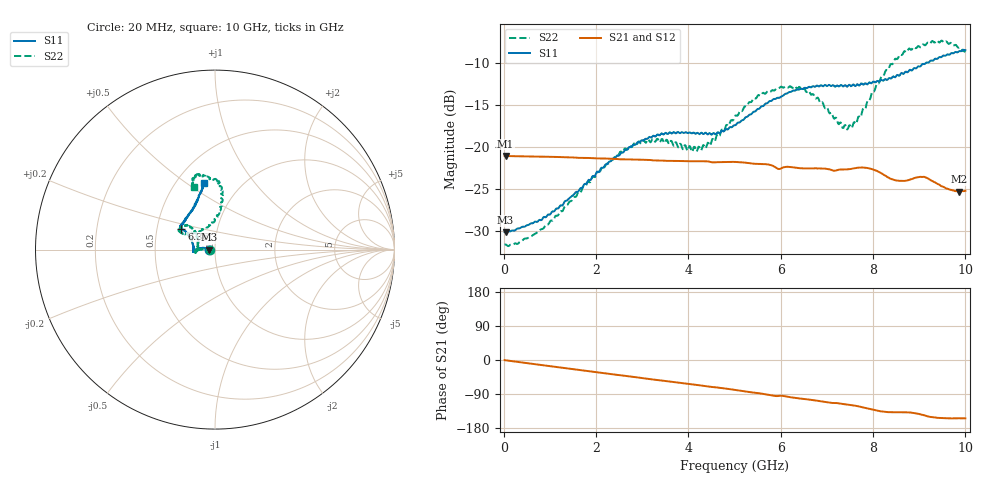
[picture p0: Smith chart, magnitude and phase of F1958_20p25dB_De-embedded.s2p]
! Integrated Device Technology
! Corporate Headquarters
! 6024 Silver Creek Valley Road
! San Jose, CA 95138  USA
! Phone:  1-408-284-8200
! Toll Free:  1-800-223-1366
! Webpage:  http://www.idt.com/
! Timing and RF Division
! 515 Groton Road, Suite 102
! Westford, MA 01886-6024
! Device:  F1958
! Description: 7-bit 0.25 dB Digital Step Attenuator
! Frequency:  0.001 -  6.000 GHz
! Package:  4x4 mm Thin QFN Plastic Package: 24 pin
! Ports:  2 RF, 12 DC
!  Pin  1  = D0
!  Pin  2  = VDD
!  Pin  3  = VMODE
!  Pin  4  = GND
!  Pin  5  = RF1  =  Port 1
!  Pin  6  = GND
!  Pin  7  = GND
!  Pin  8  = GND
!  Pin  9  = GND
!  Pin 10  = GND
!  Pin 11  = GND
!  Pin 12  = GND
!  Pin 13  = GND
!  Pin 14  = RF2  =  Port 2
!  Pin 15  = GND
!  Pin 16  = LE
!  Pin 17  = CLK
!  Pin 18  = DATA
!  Pin 19  = D6
!  Pin 20  = D5
!  Pin 21  = D4
!  Pin 22  = D3
!  Pin 23  = D2
!  Pin 24  = D1
! State:  81
! Atten State:  20.25 dB
! Voltage:  +3.30 Volts
! Current:  0.258 mA
! Data:  The device was measured on a F1958 evaluation board which has
!  individual transmission lines to the RF pins.  Data was collected
!  using a calibrated network analyzer.  The evaluation board was
!  de-embedded using Automatic Fixture Removal (AFR).
!  The reference plane is the edge of the package pin.
! Misc:
!  Action Tracker AT0419
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# GHz S dB R 50
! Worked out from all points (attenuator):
!   500 points, 20 MHz to 10 GHz, reference 50 ohm
!   highest |S21| = -21.03 dB at 40 MHz (marker M1); lowest = -25.3 dB at 9.86 GHz (marker M2)
!   lowest |S11| = -30.1 dB at 40 MHz (marker M3), VSWR 1.06, Z = 47 - j0.0438 ohm
!   |S11| at or under -10 dB: start of sweep to 9.139 GHz
!   |S22| runs from -31.7 to -7.3 dB; largest |S21 - S12| = 0.00031
!   S11 on the Smith chart (normalised r, x): 20 MHz: 0.94, -0.00; 6.36 GHz: 0.67, +0.16; 10 GHz: 0.67, +0.59
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0.02  -30.06 -178.9  -21.03 -0.4  -21.03 -0.4  -31.57 -178.6
0.04  -30.10 -179.1  -21.03 -0.7  -21.02 -0.7  -31.53 -177.9
0.32  -29.63 175.2  -21.06 -5.3  -21.06 -5.3  -31.40 177.6
0.84  -28.50 171.1  -21.11 -13.6  -21.11 -13.6  -29.70 178.0
1.7  -24.81 171.3  -21.26 -27.2  -21.25 -27.2  -24.91 176.6
2.62  -20.36 177.4  -21.42 -41.6  -21.40 -41.6  -20.15 -177.8
3.36  -18.56 -175.5  -21.58 -53.3  -21.57 -53.4  -19.27 -171.1
4.24  -18.44 -179.0  -21.65 -66.7  -21.66 -66.8  -19.96 166.7
4.64  -18.20 171.9  -21.77 -72.8  -21.78 -72.8  -18.49 148.6
5.02  -17.37 160.9  -21.74 -79.1  -21.75 -79.1  -16.21 138.1
5.58  -15.13 150.7  -21.99 -88.6  -22.00 -88.6  -13.78 138.4
6.36  -13.12 148.0  -22.44 -100.8  -22.46 -100.7  -13.04 151.5
6.68  -12.78 146.5  -22.50 -105.5  -22.52 -105.4  -13.72 152.4
7.3  -12.59 140.8  -22.64 -115.1  -22.65 -115.0  -17.05 131.1
7.5  -12.62 138.1  -22.59 -118.4  -22.60 -118.3  -17.37 112.9
7.68  -12.58 135.3  -22.42 -122.2  -22.41 -122.2  -16.37 96.1
7.92  -12.27 129.0  -22.51 -129.1  -22.51 -129.1  -14.39 86.2
8.34  -11.79 119.1  -23.60 -137.7  -23.62 -137.8  -10.65 81.7
8.68  -11.15 112.4  -23.99 -137.9  -23.98 -137.9  -8.57 86.3
9.26  -9.67 104.7  -23.93 -150.5  -23.93 -150.6  -7.49 99.2
9.86  -8.60 99.8  -25.26 -153.6  -25.29 -153.6  -8.17 108.2
10  -8.46 99.8  -25.17 -154.0  -25.20 -154.1  -8.69 109.0
